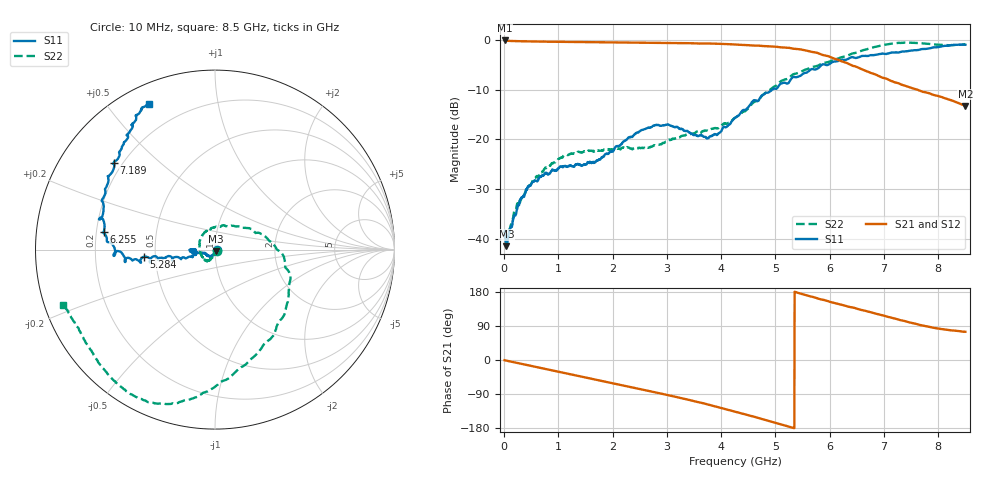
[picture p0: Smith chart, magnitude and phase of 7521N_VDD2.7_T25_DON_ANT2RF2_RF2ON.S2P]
!Agilent Technologies,E5071C,MY46417908,A.11.23
!Date: Thu Jul 30 15:13:41 2020
!Data & Calibration Information:
!Freq	S11:SOLT2(ON)	S21:SOLT2(ON)	S12:SOLT2(ON)	S22:SOLT2(ON)
!PortZ  Port1:50+j0  Port2:50+j0
!Above PortZ is port z conversion or system Z0 setting when saving the data.
!When reading, reference impedance value at option line is always used.
# Hz S dB R 50
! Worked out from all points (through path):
!   1601 points, 10 MHz to 8.5 GHz, reference 50 ohm
!   highest |S21| = -0.17 dB at 10 MHz (marker M1); lowest = -13.3 dB at 8.5 GHz (marker M2)
!   group delay of S21, straight-line fit = 98.3 ps
!   lowest |S11| = -41.4 dB at 41.84 MHz (marker M3), VSWR 1.02, Z = 50.5 - j0.712 ohm
!   |S11| at or under -10 dB: start of sweep to 4.944 GHz
!   |S22| runs from -40.4 to -0.6 dB; largest |S21 - S12| = 0.0059
!   S11 on the Smith chart (normalised r, x): 10 MHz: 1.02, -0.00; 5.284 GHz: 0.43, -0.04; 6.255 GHz: 0.23, +0.08; 7.189 GHz: 0.17, +0.36; 8.5 GHz: 0.08, +0.64
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1e7  -38.54 -11.5  -0.17 -0.6  -0.17 -0.6  -39.66 -31.9
4.18375e7  -41.40 -56.0  -0.23 -1.6  -0.23 -1.6  -40.31 -52.4
7.3675e7  -39.67 -69.3  -0.25 -2.6  -0.25 -2.6  -39.35 -69.7
2.2225e8  -34.90 -100.5  -0.31 -7.2  -0.31 -7.2  -33.91 -88.2
3.230688e8  -31.66 -105.4  -0.33 -10.3  -0.33 -10.3  -31.64 -97.4
5.353188e8  -28.46 -116.8  -0.37 -16.7  -0.37 -16.7  -28.17 -107.2
1.060638e9  -25.50 -138.9  -0.45 -32.5  -0.45 -32.5  -23.63 -117.8
1.426769e9  -25.27 -151.9  -0.51 -43.6  -0.50 -43.6  -22.67 -123.9
1.692081e9  -24.41 -162.6  -0.54 -51.7  -0.54 -51.7  -22.23 -124.1
2.1325e9  -21.21 -167.3  -0.59 -65.3  -0.59 -65.2  -21.90 -136.0
2.843538e9  -17.11 -175.8  -0.68 -87.2  -0.67 -87.2  -21.08 167.0
3.750906e9  -19.74 -170.2  -0.78 -117.2  -0.78 -117.2  -18.25 92.6
4.255e9  -15.67 -163.5  -0.97 -136.1  -0.98 -136.1  -15.67 53.6
4.7644e9  -11.12 -170.5  -1.28 -156.3  -1.28 -156.3  -11.11 17.4
5.284412e9  -7.96 -174.3  -1.73 -177.6  -1.73 -177.7  -7.31 -16.9
5.671769e9  -5.89 -172.9  -2.46 167.0  -2.46 167.0  -5.47 -44.4
6.255456e9  -4.05 170.8  -4.46 144.7  -4.44 144.3  -3.44 -77.8
6.743631e9  -3.13 151.5  -6.62 126.4  -6.56 126.0  -1.72 -96.3
7.088538e9  -2.74 140.3  -8.06 113.3  -8.03 113.1  -0.90 -107.3
7.189356e9  -2.60 139.3  -8.53 109.9  -8.48 109.8  -0.74 -111.1
7.597938e9  -2.12 129.8  -9.97 95.0  -9.96 95.0  -0.67 -125.6
8.5e9  -1.03 114.3  -13.29 74.5  -13.38 73.9  -0.91 -159.8
